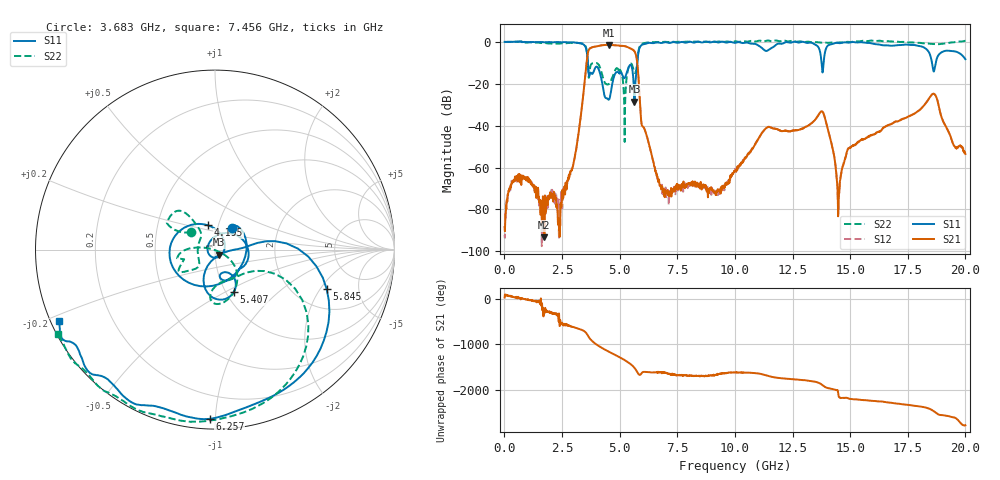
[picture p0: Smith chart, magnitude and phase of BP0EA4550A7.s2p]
! 9/17/2020 12:53:35 PM
! C:\ANRITSUVNA\DATA\MLO\SAMPLES\RAYTHEOM BP\17373_20GH_91720 .S2P
! CHANNEL.1
! TR.MEASUREMENT
! CORRECTED.DATA
# GHZ S RI R 50.0
! FREQ.GHZ  S11RE  S11IM  S31RE  S31IM  S13RE  S13IM  S33RE  S33IM
!; PortSelection: Port_13
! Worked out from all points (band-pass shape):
!   1601 points, 10 MHz to 20 GHz, reference 50 ohm
!   highest |S21| = -1.43 dB at 4.545 GHz (marker M1); lowest = -93.3 dB at 1.734 GHz (marker M2)
!   |S21| within 3 dB of the highest: 3.641 GHz to 5.636 GHz (1.995 GHz wide, 43 % of centre)
!   lowest |S11| = -28.5 dB at 5.645 GHz (marker M3), VSWR 1.08, Z = 52.3 - j3.06 ohm
!   |S11| at or under -10 dB: 3.622 GHz to 5.764 GHz (2.143 GHz wide, 45.7 % of centre); 13.76 GHz to 13.85 GHz (87.94 MHz wide, 0.637 % of centre); 18.55 GHz to 18.71 GHz (161.4 MHz wide, 0.866 % of centre)
!   |S22| runs from -47.8 to 0.7 dB; largest |S21 - S12| = 0.0018
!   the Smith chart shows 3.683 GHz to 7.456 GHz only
!   S11 on the Smith chart (normalised r, x): 3.683 GHz: 1.17, +0.29; 4.195 GHz: 0.89, +0.25; 5.407 GHz: 1.09, -0.55; 5.845 GHz: 2.94, -2.31; 6.257 GHz: 0.06, -0.97; 7.456 GHz: 0.02, -0.22
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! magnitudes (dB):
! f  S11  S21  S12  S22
! 10 MHz  0.0  -88.4  -92.2  0.0
! 672.2 MHz  0.1  -64.6  -63.9  0.2
! 1.734 GHz  -0.2  -93.3  -87.4  -0.5
! 2.396 GHz  -0.2  -93.1  -78.0  -0.8
! 3.346 GHz  -0.8  -32.7  -32.7  -0.8
! 3.683 GHz  -16.3  -3.4  -3.4  -15.7
! 4.195 GHz  -17.1  -1.7  -1.7  -13.8
! 4.545 GHz  -27.4  -1.4  -1.4  -20.0
! 5.407 GHz  -11.7  -2.8  -2.8  -11.6
! 5.645 GHz  -28.5  -4.6  -4.6  -14.7
! 5.845 GHz  -3.6  -21.7  -21.7  -3.0
! 6.257 GHz  -0.5  -48.2  -48.2  -0.3
! 6.682 GHz  -0.3  -66.3  -66.0  -0.1
! 7.456 GHz  -0.4  -68.6  -69.8  0.0
! 10.01 GHz  -0.4  -61.4  -60.9  0.2
! 13.34 GHz  -0.5  -38.7  -38.6  -0.2
! 13.87 GHz  -8.1  -34.8  -34.8  -0.3
! 14.5 GHz  -0.6  -75.2  -75.4  -0.3
! 14.95 GHz  -0.4  -50.6  -50.7  0.0
! 16.68 GHz  -1.8  -39.7  -39.6  0.3
! 18.63 GHz  -14.2  -24.8  -24.8  -1.0
! 20 GHz  -8.3  -53.5  -53.1  0.5
